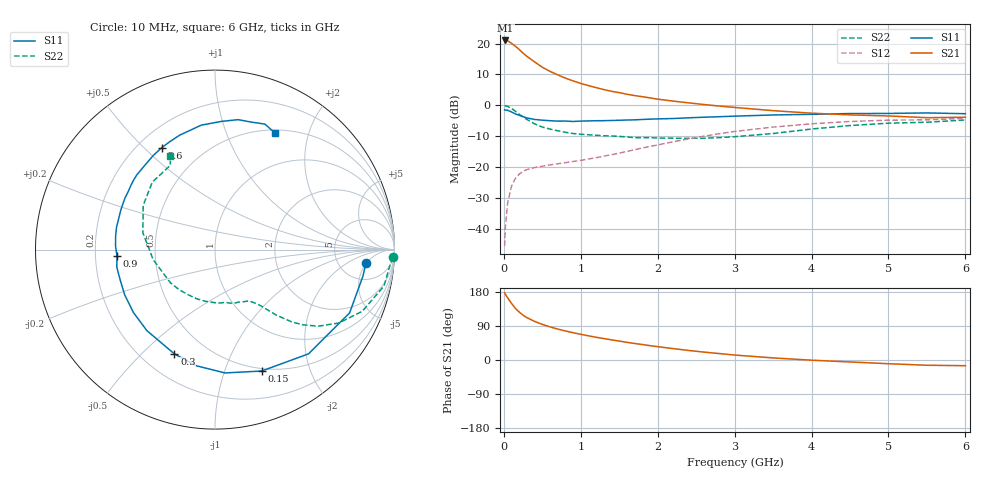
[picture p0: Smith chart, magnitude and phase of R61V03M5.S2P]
! SIEMENS Small Signal Semiconductors
! BFR193
! Si NPN RF Bipolar Junction Transistor in SOT23
! VCE = 1 V  IC = 3.5 mA
! Common Emitter S-Parameters:  May  1996
# GHz  S  MA  R  50
!  f  S11  S21  S12  S22
! GHz  MAG  ANG  MAG  ANG  MAG  ANG  MAG  ANG
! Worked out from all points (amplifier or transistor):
!   36 points, 10 MHz to 6 GHz, reference 50 ohm
!   highest |S21| = 21.0 dB at 20 MHz (marker M1)
!   |S21| within 3 dB of that: start of sweep to 202.6 MHz
!   unconditionally stable (mu >= 1): 962.8 MHz to 2.183 GHz
!   at 250 MHz: K = 0.34, MSG = 19.2 dB, |S12| = -21.5 dB
!   at 1.4 GHz: K = 1.10, MAG = 8.4 dB, |S12| = -16.0 dB
!   at 6 GHz: K = 1.00, MSG = 0.2 dB, |S12| = -4.2 dB
!   S11 on the Smith chart (normalised r, x): 10 MHz: 9, -5; 150 MHz: 0.47, -1.35; 300 MHz: 0.33, -0.63; 900 MHz: 0.29, -0.03; 2.6 GHz: 0.29, +0.57; 6 GHz: 0.53, +1.50
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0.01  0.8441 -5.1  11.15 177.1  0.0052 86.0  0.993 -2.4
0.02  0.8377 -10.1  11.27 173.3  0.0107 85.9  0.9798 -4.8
0.05  0.8287 -25.2  11.12 163.8  0.0263 75.9  0.9631 -12.2
0.1  0.7803 -48.1  10.12 149.4  0.049 65.8  0.8899 -22.7
0.15  0.7247 -69.0  9.089 136.1  0.0653 56.8  0.8015 -30.7
0.2  0.6894 -85.4  8.031 126.4  0.0766 50.7  0.7158 -36.6
0.25  0.6554 -99.2  7.004 118.4  0.0845 45.8  0.6454 -40.5
0.3  0.6234 -111.3  6.231 111.7  0.0908 43.2  0.5897 -43.2
0.4  0.5899 -130.0  5.054 101.9  0.0978 39.8  0.5004 -46.9
0.5  0.574 -142.3  4.143 94.0  0.1028 38.4  0.4439 -49.0
0.6  0.5629 -153.3  3.552 87.4  0.1081 38.6  0.4119 -50.4
0.7  0.5546 -162.5  3.121 81.6  0.1126 39.4  0.3863 -52.0
0.9  0.5471 -176.1  2.488 72.0  0.1229 42.9  0.3486 -55.8
1.1  0.5588 172.2  2.088 63.8  0.1345 46.1  0.3327 -60.5
1.3  0.5635 162.4  1.799 56.5  0.15 49.0  0.3208 -65.7
1.6  0.5777 150.4  1.511 46.6  0.1787 52.5  0.3072 -75.6
2.2  0.6108 130.0  1.171 30.1  0.2564 53.0  0.293 -100.2
2.6  0.6411 117.5  1.03 20.9  0.3158 49.5  0.2926 -120.8
3.5  0.6976 96.3  0.819 5.5  0.4436 35.5  0.349 -170.7
4.5  0.7352 80.0  0.7 -5.2  0.547 18.1  0.4701 148.3
5.5  0.7526 68.3  0.63 -13.9  0.5813 1.5  0.5313 117.9
6  0.731 63.0  0.641 -15.0  0.6148 -3.2  0.5793 115.5
